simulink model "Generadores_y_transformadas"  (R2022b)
settings: Solver=ode4  StartTime=0.0  StopTime=0.1  FixedStep=1e-6  RelTol=1e-3
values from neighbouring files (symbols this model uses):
  f_AC = 60    [Generadores_y_tranformadas.m]
  Fase_A = 0    [Generadores_y_tranformadas.m]
  Fase_B = -120    [Generadores_y_tranformadas.m]
  Fase_C = 120    [Generadores_y_tranformadas.m]
  L_1 = 4.1e-3    (= 0.0041)    [Generadores_y_tranformadas.m]    (also in LQR_Sin_Integral.m; LQR_Con_Integral.m; Modal_Integral.m; Sistema_no_lineal_Modal.m)
  L_2 = 5.3e-3    (= 0.0053)    [Generadores_y_tranformadas.m]    (also in Sistema_no_lineal_Modal.m; Sistema_no_lineal_LQR.m; Sistema_control_no_lineal_LQR.m; Sistema_control_no_lineal_Modal.m)
  R_1 = 284e-3    (= 0.284)    [Generadores_y_tranformadas.m]    (also in LQR_Sin_Integral.m; LQR_Con_Integral.m; Modal_Integral.m; Sistema_no_lineal_Modal.m)
  R_2 = 330e-3    (= 0.33)    [Generadores_y_tranformadas.m]    (also in Sistema_no_lineal_Modal.m; Sistema_no_lineal_LQR.m; Sistema_control_no_lineal_LQR.m; Sistema_control_no_lineal_Modal.m)
  v_pico = v_RMS*sqrt(2)    [Generadores_y_tranformadas.m]
libraries: spsACVoltageSourceLib x6, spsGroundLib x6, spsCurrentMeasurementLib x6, spsVoltageMeasurementLib x6, spsSeriesRLCBranchLib x6, spsAlphaBetaZerotodq0Lib x4, spsabctoAlphaBetaZeroLib x4, spsAlphaBetaZerotoabcLib x1, spsdq0toAlphaBetaZeroLib x1, spspowerguiLib x1

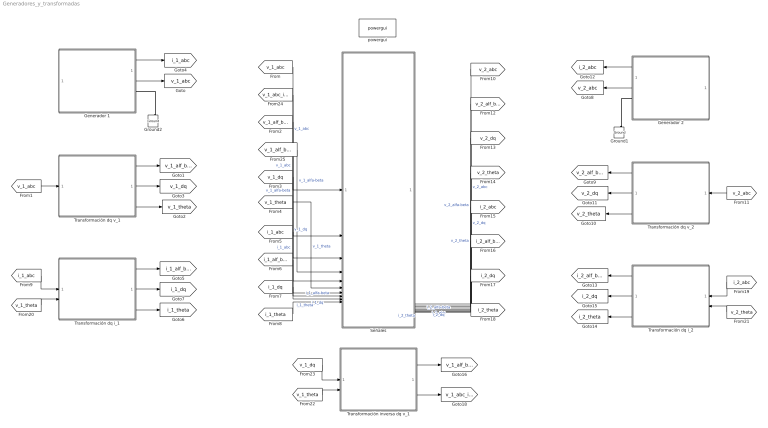
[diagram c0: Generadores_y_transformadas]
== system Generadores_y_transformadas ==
  Generador 1 : Subsystem
  Generador 2 : Subsystem
  Ground1 : spsGroundLib/Ground  LConnTagsString=a
  Ground2 : spsGroundLib/Ground  LConnTagsString=a
  Señales : Subsystem
  Transformación dq i_1 : Subsystem
  Transformación dq i_2 : Subsystem
  Transformación dq v_1 : Subsystem
  Transformación dq v_2 : Subsystem
  Transformación inversa dq v_1 : Subsystem
  powergui : spspowerguiLib/powergui  Priority=1  SimulationMode=Continuous  SampleTime=5e-6  frequency=Frecuencia_fuente  Iterations=50  frequencyindice=60  Pbase=100e6  ErrMax=1e-4  UnitsV=kV  UnitsW=MW  buscounter=0  FunctionMessages=off  echomessages=off  EnableUseOfTLC=off  CurrentSourceSwitches=off  DisableSnubberDevices=off  DisableRonSwitches=off  DisableVfSwitches=off  DisplayEquations=off  AutomaticDiscreteSolvers=off  SolverType=Tustin/Backward Euler (TBE)  Interpol=off  ExternalGateDelay=off  methode=off  Ts=100  x0status=blocks  SPID=on  SwTol=0  HookPort=off  NonlinearTolerance=1e-4  nMaxIteration=100  ContinueOnMaxIteration=off  RestoreLinks=warning  ResistiveCurrentMeasurement=off  Frange=[0:2:500]  Ylog=off  Xlog=on  ShowGrid=off  save=off  variable=ZData  structure=0  ZoomFFT=off  StartTime=0.0  cycles=1  DisplayStyle=1  fundamental=60  FreqAxis=off  MaxFrequency=1000  frequencyindicesteady=1  RmsSteady=1  display=off
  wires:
  Transformación dq i_1/1(i_1_alfa-beta) -> [i_1_alf_bet]
  Transformación dq i_1/3(Ángulo theta i_1) -> [i_1_theta]
  Transformación dq i_1/2(i_1_dq) -> [i_1_dq]
  Transformación dq v_1/1(v_1_alfa-beta) -> [v_1_alf_bet]
  [v_1_abc] -> Transformación dq v_1/1(v_1_abc)
  Transformación dq v_1/3(Ángulo theta v_1) -> [v_1_theta]
  Transformación dq v_1/2(v_1_dq) -> [v_1_dq]
  [i_1_abc] -> Transformación dq i_1/1(i_1_abc)
  Generador 1/1(i_1_abc) -> [i_1_abc]
  Generador 1/2(v_1_abc) -> [v_1_abc]
  [v_1_abc] -> Señales/1(v_1_abc)  "v_1_abc"
  [v_1_alf_bet] -> Señales/3(v_1_alfa-beta)  "v_1_alfa-beta"
  [v_1_dq] -> Señales/5(v_1_dq)  "v_1_dq"
  [v_1_theta] -> Señales/6(v_1_theta)  "v_1_theta"
  [i_1_abc] -> Señales/7(i_1_abc)  "i_1_abc"
  [i_1_alf_bet] -> Señales/8(i_1_alfa-beta)  "i_1_alfa-beta"
  [i_1_dq] -> Señales/9(i_1_dq)  "i_1_dq"
  [i_1_theta] -> Señales/10(i_1_theta)  "i_1_theta"
  Generador 2/2(v_2_abc) -> [v_2_abc]
  Generador 2/1(i_2_abc) -> [i_2_abc]
  [i_2_abc] -> Transformación dq i_2/1(i_2_abc)
  Transformación dq v_2/2(v_2_dq) -> [v_2_dq]
  Transformación dq v_2/3(Ángulo theta v_2) -> [v_2_theta]
  [v_2_abc] -> Transformación dq v_2/1(v_2_abc)
  Transformación dq v_2/1(v_2_alfa-beta) -> [v_2_alf_bet]
  Transformación dq i_2/2(i_2_dq) -> [i_2_dq]
  Transformación dq i_2/3(Ángulo theta i_2) -> [i_2_theta]
  Transformación dq i_2/1(i_2_alfa-beta) -> [i_2_alf_bet]
  [v_2_abc] -> Señales/11(v_2_abc)  "v_2_abc"
  [v_2_alf_bet] -> Señales/12(v_2_alfa-beta)  "v_2_alfa-beta"
  [v_2_dq] -> Señales/13(v_2_dq)  "v_2_dq"
  [v_2_theta] -> Señales/14(v_2_theta)  "v_2_theta"
  [i_2_abc] -> Señales/15(i_2_abc)  "i_2_abc"
  [i_2_alf_bet] -> Señales/16(i_2_alfa-beta)  "i_2_alfa-beta"
  [i_2_dq] -> Señales/17(i_2_dq)  "i_2_dq"
  [i_2_theta] -> Señales/18(i_2_theta)  "i_2_theta"
  [v_1_theta] -> Transformación dq i_1/2(Ángulo theta v_1)
  [v_2_theta] -> Transformación dq i_2/2(Ángulo theta v_2)
  [v_1_dq] -> Transformación inversa dq v_1/1(v_1_dq)
  Transformación inversa dq v_1/2(v_1_abc) -> [v_1_abc_inv]
  [v_1_theta] -> Transformación inversa dq v_1/2(Ángulo theta v_1)
  Transformación inversa dq v_1/1(v_1_alfa-beta) -> [v_1_alf_bet_inv]
  [v_1_abc_inv] -> Señales/2(v_1_abc_inv)  "v_1_abc"
  [v_1_alf_bet_inv] -> Señales/4(v_1_alfa-beta_inv)  "v_1_alfa-beta"
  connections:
  Ground2/LConn1 -- Generador 1/RConn1
  Ground1/LConn1 -- Generador 2/RConn1

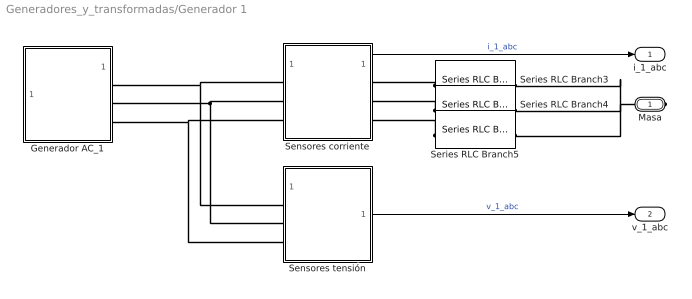
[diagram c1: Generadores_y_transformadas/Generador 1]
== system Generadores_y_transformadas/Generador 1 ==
  Generador AC_1 : Subsystem
  Sensores corriente : Subsystem
  Sensores tensión : Subsystem
  Series RLC Branch3 : spsSeriesRLCBranchLib/Series RLC Branch  LConnTagsString=__new0  RConnTagsString=__new0  BranchType=RL  Resistance=R_1  Inductance=L_1  SetiL0=off  InitialCurrent=0  Capacitance=1e-6  Setx0=off  InitialVoltage=0  Measurements=None
  Series RLC Branch4 : spsSeriesRLCBranchLib/Series RLC Branch  LConnTagsString=__new0  RConnTagsString=__new0  BranchType=RL  Resistance=R_1  Inductance=L_1  SetiL0=off  InitialCurrent=0  Capacitance=1e-6  Setx0=off  InitialVoltage=0  Measurements=None
  Series RLC Branch5 : spsSeriesRLCBranchLib/Series RLC Branch  LConnTagsString=__new0  RConnTagsString=__new0  BranchType=RL  Resistance=R_1  Inductance=L_1  SetiL0=off  InitialCurrent=0  Capacitance=1e-6  Setx0=off  InitialVoltage=0  Measurements=None
  Masa : PMIOPort  Side=Right
  i_1_abc : Outport
  v_1_abc : Outport  Port=2
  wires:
  Sensores tensión/1(v_1_abc) -> v_1_abc/1  "v_1_abc"
  Sensores corriente/1(i_1_abc) -> i_1_abc/1  "i_1_abc"
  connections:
  Masa/RConn1 -- Series RLC Branch5/RConn1 -- Series RLC Branch4/RConn1 -- Series RLC Branch3/RConn1
  Sensores tensión/LConn2 -- Generador AC_1/RConn2 -- Sensores corriente/LConn2
  Generador AC_1/RConn1 -- Sensores corriente/LConn1 -- Sensores tensión/LConn1
  Sensores tensión/LConn3 -- Generador AC_1/RConn3 -- Sensores corriente/LConn3
  Series RLC Branch4/LConn1 -- Sensores corriente/RConn2
  Series RLC Branch3/LConn1 -- Sensores corriente/RConn1
  Series RLC Branch5/LConn1 -- Sensores corriente/RConn3

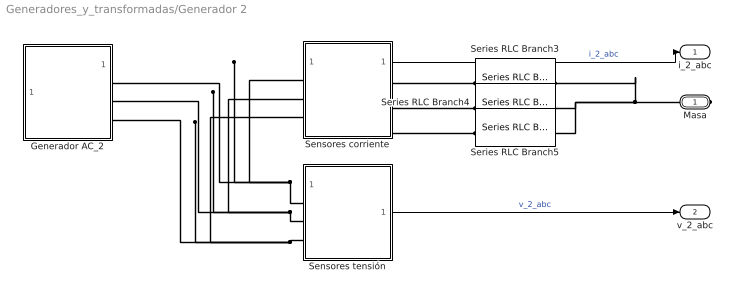
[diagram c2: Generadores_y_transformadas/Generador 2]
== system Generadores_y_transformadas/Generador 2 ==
  Generador AC_2 : Subsystem
  Sensores corriente : Subsystem
  Sensores tensión : Subsystem
  Series RLC Branch3 : spsSeriesRLCBranchLib/Series RLC Branch  LConnTagsString=__new0  RConnTagsString=__new0  BranchType=RL  Resistance=R_2  Inductance=L_2  SetiL0=off  InitialCurrent=0  Capacitance=1e-6  Setx0=off  InitialVoltage=0  Measurements=None
  Series RLC Branch4 : spsSeriesRLCBranchLib/Series RLC Branch  LConnTagsString=__new0  RConnTagsString=__new0  BranchType=RL  Resistance=R_2  Inductance=L_2  SetiL0=off  InitialCurrent=0  Capacitance=1e-6  Setx0=off  InitialVoltage=0  Measurements=None
  Series RLC Branch5 : spsSeriesRLCBranchLib/Series RLC Branch  LConnTagsString=__new0  RConnTagsString=__new0  BranchType=RL  Resistance=R_2  Inductance=L_2  SetiL0=off  InitialCurrent=0  Capacitance=1e-6  Setx0=off  InitialVoltage=0  Measurements=None
  Masa : PMIOPort  Side=Right
  i_2_abc : Outport
  v_2_abc : Outport  Port=2
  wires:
  Sensores corriente/1(i_2_abc) -> i_2_abc/1  "i_2_abc"
  Sensores tensión/1(v_2_abc) -> v_2_abc/1  "v_2_abc"
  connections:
  Sensores tensión/LConn1 -- Generador AC_2/RConn1 -- Sensores corriente/LConn1
  Sensores tensión/LConn3 -- Generador AC_2/RConn3 -- Sensores corriente/LConn3
  Sensores corriente/RConn3 -- Series RLC Branch5/LConn1
  Sensores corriente/RConn2 -- Series RLC Branch4/LConn1
  Sensores corriente/RConn1 -- Series RLC Branch3/LConn1
  Masa/RConn1 -- Series RLC Branch5/RConn1 -- Series RLC Branch3/RConn1 -- Series RLC Branch4/RConn1
  Sensores tensión/LConn2 -- Generador AC_2/RConn2 -- Sensores corriente/LConn2

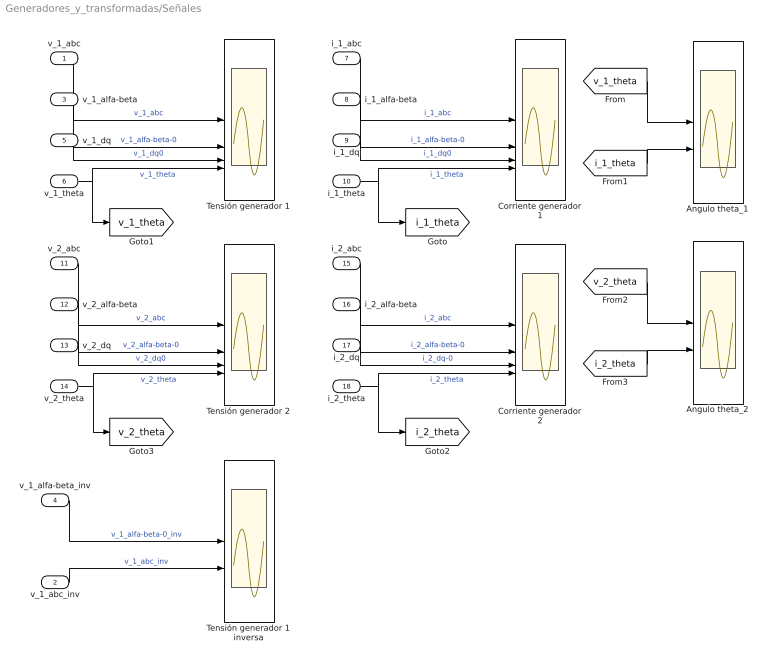
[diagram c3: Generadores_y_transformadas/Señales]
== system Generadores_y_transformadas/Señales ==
  v_1_abc : Inport
  v_1_abc_inv : Inport  Port=2
  v_1_alfa-beta : Inport  Port=3
  v_1_alfa-beta_inv : Inport  Port=4
  v_1_dq : Inport  Port=5
  v_1_theta : Inport  Port=6
  i_1_abc : Inport  Port=7
  i_1_alfa-beta : Inport  Port=8
  i_1_dq : Inport  Port=9
  i_1_theta : Inport  Port=10
  v_2_abc : Inport  Port=11
  v_2_alfa-beta : Inport  Port=12
  v_2_dq : Inport  Port=13
  v_2_theta : Inport  Port=14
  i_2_abc : Inport  Port=15
  i_2_alfa-beta : Inport  Port=16
  i_2_dq : Inport  Port=17
  i_2_theta : Inport  Port=18
  Angulo theta_1 : Scope  NumInputPorts=2
  Angulo theta_2 : Scope  NumInputPorts=2
  Corriente generador 1 : Scope  NumInputPorts=4
  Corriente generador 2 : Scope  NumInputPorts=4
  Tensión generador 1 : Scope  NumInputPorts=4
  Tensión generador 1 inversa : Scope  NumInputPorts=2
  Tensión generador 2 : Scope  NumInputPorts=4
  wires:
  v_1_alfa-beta/1 -> Tensión generador 1/2  "v_1_alfa-beta-0"
  v_1_theta/1 -> Tensión generador 1/4, [v_1_theta]  "v_1_theta"
  v_1_dq/1 -> Tensión generador 1/3  "v_1_dq0"
  v_1_abc/1 -> Tensión generador 1/1  "v_1_abc"
  i_1_abc/1 -> Corriente generador 1/1  "i_1_abc"
  i_1_dq/1 -> Corriente generador 1/3  "i_1_dq0"
  i_1_theta/1 -> Corriente generador 1/4, [i_1_theta]  "i_1_theta"
  i_1_alfa-beta/1 -> Corriente generador 1/2  "i_1_alfa-beta-0"
  v_2_abc/1 -> Tensión generador 2/1  "v_2_abc"
  v_2_alfa-beta/1 -> Tensión generador 2/2  "v_2_alfa-beta-0"
  v_2_dq/1 -> Tensión generador 2/3  "v_2_dq0"
  v_2_theta/1 -> Tensión generador 2/4, [v_2_theta]  "v_2_theta"
  i_2_theta/1 -> Corriente generador 2/4, [i_2_theta]  "i_2_theta"
  i_2_dq/1 -> Corriente generador 2/3  "i_2_dq-0"
  i_2_alfa-beta/1 -> Corriente generador 2/2  "i_2_alfa-beta-0"
  i_2_abc/1 -> Corriente generador 2/1  "i_2_abc"
  [v_1_theta] -> Angulo theta_1/1
  [i_1_theta] -> Angulo theta_1/2
  [i_2_theta] -> Angulo theta_2/2
  [v_2_theta] -> Angulo theta_2/1
  v_1_alfa-beta_inv/1 -> Tensión generador 1 inversa/1  "v_1_alfa-beta-0_inv"
  v_1_abc_inv/1 -> Tensión generador 1 inversa/2  "v_1_abc_inv"

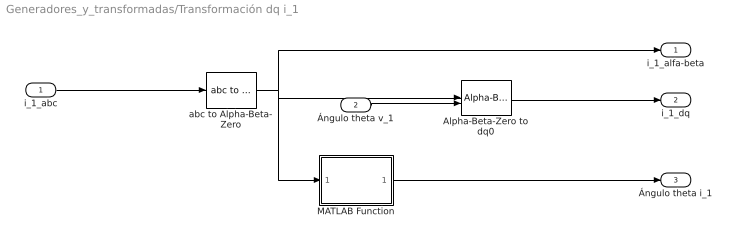
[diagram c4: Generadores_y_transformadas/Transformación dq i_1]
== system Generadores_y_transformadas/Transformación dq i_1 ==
  i_1_abc : Inport
  Ángulo theta v_1 : Inport  Port=2
  Alpha-Beta-Zero to dq0 : spsAlphaBetaZerotodq0Lib/Alpha-Beta-Zero to dq0  Alignment=Aligned with phase A axis
  MATLAB Function : MATLAB Function  TreatAsAtomicUnit=on
  abc to Alpha-Beta-Zero : spsabctoAlphaBetaZeroLib/abc to Alpha-Beta-Zero
  i_1_alfa-beta : Outport
  i_1_dq : Outport  Port=2
  Ángulo theta i_1 : Outport  Port=3
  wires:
  i_1_abc/1 -> abc to Alpha-Beta-Zero/1
  MATLAB Function/1(angulo) -> Ángulo theta i_1/1
  Alpha-Beta-Zero to dq0/1 -> i_1_dq/1
  abc to Alpha-Beta-Zero/1 -> i_1_alfa-beta/1, Alpha-Beta-Zero to dq0/1, MATLAB Function/1(u)
  Ángulo theta v_1/1 -> Alpha-Beta-Zero to dq0/2

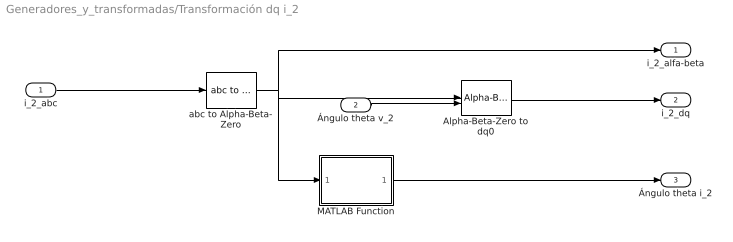
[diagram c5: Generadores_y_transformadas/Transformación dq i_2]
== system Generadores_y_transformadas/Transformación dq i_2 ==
  i_2_abc : Inport
  Ángulo theta v_2 : Inport  Port=2
  Alpha-Beta-Zero to dq0 : spsAlphaBetaZerotodq0Lib/Alpha-Beta-Zero to dq0  Alignment=Aligned with phase A axis
  MATLAB Function : MATLAB Function  TreatAsAtomicUnit=on
  abc to Alpha-Beta-Zero : spsabctoAlphaBetaZeroLib/abc to Alpha-Beta-Zero
  i_2_alfa-beta : Outport
  i_2_dq : Outport  Port=2
  Ángulo theta i_2 : Outport  Port=3
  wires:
  abc to Alpha-Beta-Zero/1 -> MATLAB Function/1(u), Alpha-Beta-Zero to dq0/1, i_2_alfa-beta/1
  Alpha-Beta-Zero to dq0/1 -> i_2_dq/1
  MATLAB Function/1(angulo) -> Ángulo theta i_2/1
  i_2_abc/1 -> abc to Alpha-Beta-Zero/1
  Ángulo theta v_2/1 -> Alpha-Beta-Zero to dq0/2

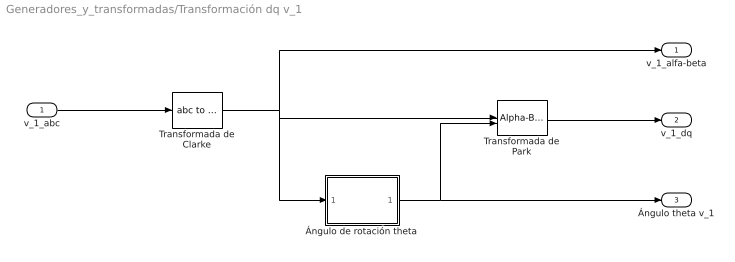
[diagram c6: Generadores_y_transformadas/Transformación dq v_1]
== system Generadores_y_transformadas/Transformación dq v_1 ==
  v_1_abc : Inport
  Transformada de Clarke : spsabctoAlphaBetaZeroLib/abc to Alpha-Beta-Zero
  Transformada de Park : spsAlphaBetaZerotodq0Lib/Alpha-Beta-Zero to dq0  Alignment=Aligned with phase A axis
  Ángulo de rotación theta : MATLAB Function  TreatAsAtomicUnit=on
  v_1_alfa-beta : Outport
  v_1_dq : Outport  Port=2
  Ángulo theta v_1 : Outport  Port=3
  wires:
  v_1_abc/1 -> Transformada de Clarke/1
  Ángulo de rotación theta/1(angulo) -> Ángulo theta v_1/1, Transformada de Park/2
  Transformada de Park/1 -> v_1_dq/1
  Transformada de Clarke/1 -> v_1_alfa-beta/1, Transformada de Park/1, Ángulo de rotación theta/1(u)

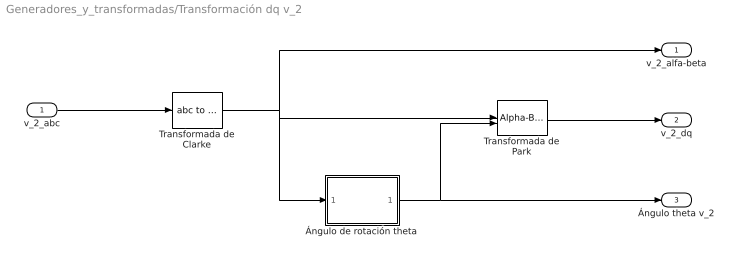
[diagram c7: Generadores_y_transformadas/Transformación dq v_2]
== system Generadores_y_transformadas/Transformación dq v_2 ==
  v_2_abc : Inport
  Transformada de Clarke : spsabctoAlphaBetaZeroLib/abc to Alpha-Beta-Zero
  Transformada de Park : spsAlphaBetaZerotodq0Lib/Alpha-Beta-Zero to dq0  Alignment=Aligned with phase A axis
  Ángulo de rotación theta : MATLAB Function  TreatAsAtomicUnit=on
  v_2_alfa-beta : Outport
  v_2_dq : Outport  Port=2
  Ángulo theta v_2 : Outport  Port=3
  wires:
  Transformada de Clarke/1 -> Ángulo de rotación theta/1(u), Transformada de Park/1, v_2_alfa-beta/1
  Transformada de Park/1 -> v_2_dq/1
  Ángulo de rotación theta/1(angulo) -> Transformada de Park/2, Ángulo theta v_2/1
  v_2_abc/1 -> Transformada de Clarke/1

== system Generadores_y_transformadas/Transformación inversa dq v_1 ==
  v_1_dq : Inport
  Ángulo theta v_1 : Inport  Port=2
  Alpha-Beta-Zero to abc : spsAlphaBetaZerotoabcLib/Alpha-Beta-Zero to abc
  dq0 to Alpha-Beta-Zero : spsdq0toAlphaBetaZeroLib/dq0 to Alpha-Beta-Zero  Alignment=90 degrees behind phase A axis
  v_1_alfa-beta : Outport
  v_1_abc : Outport  Port=2
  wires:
  v_1_dq/1 -> dq0 to Alpha-Beta-Zero/1
  Alpha-Beta-Zero to abc/1 -> v_1_abc/1
  dq0 to Alpha-Beta-Zero/1 -> v_1_alfa-beta/1, Alpha-Beta-Zero to abc/1
  Ángulo theta v_1/1 -> dq0 to Alpha-Beta-Zero/2

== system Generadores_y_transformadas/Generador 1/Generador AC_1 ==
  Generador fase A : spsACVoltageSourceLib/AC Voltage Source  Amplitude=v_pico  Phase=Fase_A  Frequency=f_AC  SampleTime=0  Measurements=Voltage  BusType=swing  Pref=10e3  Qref=0  Qmin=-inf  Qmax=+inf
  Generador fase B : spsACVoltageSourceLib/AC Voltage Source  Amplitude=v_pico  Phase=Fase_B  Frequency=f_AC  SampleTime=0  Measurements=Voltage  BusType=swing  Pref=10e3  Qref=0  Qmin=-inf  Qmax=+inf
  Generador fase C : spsACVoltageSourceLib/AC Voltage Source  Amplitude=v_pico  Phase=Fase_C  Frequency=f_AC  SampleTime=0  Measurements=Voltage  BusType=swing  Pref=10e3  Qref=0  Qmin=-inf  Qmax=+inf
  Ground3 : spsGroundLib/Ground  LConnTagsString=a
  Fase A : PMIOPort  Side=Right
  Fase B : PMIOPort  Port=2  Side=Right
  Fase C : PMIOPort  Port=3  Side=Right
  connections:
  Generador fase C/RConn1 -- Fase C/RConn1
  Generador fase B/RConn1 -- Fase B/RConn1
  Generador fase A/RConn1 -- Fase A/RConn1
  Generador fase B/LConn1 -- Generador fase C/LConn1 -- Ground3/LConn1 -- Generador fase A/LConn1

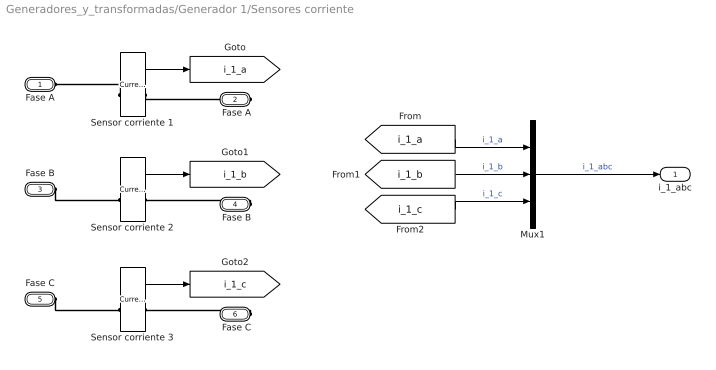
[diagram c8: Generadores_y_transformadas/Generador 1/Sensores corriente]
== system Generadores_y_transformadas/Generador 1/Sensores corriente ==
  Mux1 : Mux  Inputs=3
  Sensor corriente 1 : spsCurrentMeasurementLib/Current Measurement  PhasorSimulation=off  OutputType=Complex  PSBequivalent=0
  Sensor corriente 2 : spsCurrentMeasurementLib/Current Measurement  PhasorSimulation=off  OutputType=Complex  PSBequivalent=0
  Sensor corriente 3 : spsCurrentMeasurementLib/Current Measurement  PhasorSimulation=off  OutputType=Complex  PSBequivalent=0
  Fase A : PMIOPort  Side=Left
  " Fase A" : PMIOPort  Port=2  Side=Right
  Fase B : PMIOPort  Port=3  Side=Left
  " Fase B" : PMIOPort  Port=4  Side=Right
  Fase C : PMIOPort  Port=5  Side=Left
  " Fase C" : PMIOPort  Port=6  Side=Right
  i_1_abc : Outport
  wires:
  Mux1/1 -> i_1_abc/1  "i_1_abc"
  Sensor corriente 1/1 -> [i_1_a]
  [i_1_a] -> Mux1/1  "i_1_a"
  Sensor corriente 2/1 -> [i_1_b]
  [i_1_b] -> Mux1/2  "i_1_b"
  Sensor corriente 3/1 -> [i_1_c]
  [i_1_c] -> Mux1/3  "i_1_c"
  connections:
  Fase C/RConn1 -- Sensor corriente 3/LConn1
  " Fase B"/RConn1 -- Sensor corriente 2/RConn1
  Fase B/RConn1 -- Sensor corriente 2/LConn1
  Sensor corriente 1/LConn1 -- Fase A/RConn1
  " Fase C"/RConn1 -- Sensor corriente 3/RConn1
  Sensor corriente 1/RConn1 -- " Fase A"/RConn1

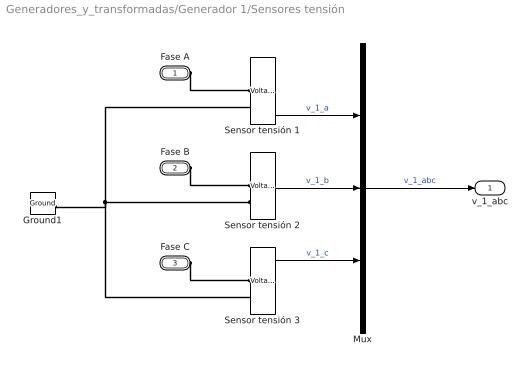
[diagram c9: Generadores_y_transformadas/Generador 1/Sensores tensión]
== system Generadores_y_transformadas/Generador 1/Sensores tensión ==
  Ground1 : spsGroundLib/Ground  LConnTagsString=a
  Mux : Mux  Inputs=3
  Sensor tensión 1 : spsVoltageMeasurementLib/Voltage Measurement  PhasorSimulation=off  OutputType=Complex  PSBequivalent=0
  Sensor tensión 2 : spsVoltageMeasurementLib/Voltage Measurement  PhasorSimulation=off  OutputType=Complex  PSBequivalent=0
  Sensor tensión 3 : spsVoltageMeasurementLib/Voltage Measurement  PhasorSimulation=off  OutputType=Complex  PSBequivalent=0
  Fase A : PMIOPort  Side=Left
  Fase B : PMIOPort  Port=2  Side=Left
  Fase C : PMIOPort  Port=3  Side=Left
  v_1_abc : Outport
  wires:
  Mux/1 -> v_1_abc/1  "v_1_abc"
  Sensor tensión 2/1 -> Mux/2  "v_1_b"
  Sensor tensión 3/1 -> Mux/3  "v_1_c"
  Sensor tensión 1/1 -> Mux/1  "v_1_a"
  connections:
  Fase B/RConn1 -- Sensor tensión 2/LConn1
  Fase C/RConn1 -- Sensor tensión 3/LConn1
  Fase A/RConn1 -- Sensor tensión 1/LConn1
  Sensor tensión 2/LConn2 -- Sensor tensión 1/LConn2 -- Ground1/LConn1 -- Sensor tensión 3/LConn2

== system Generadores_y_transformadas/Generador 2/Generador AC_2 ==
  Generador fase A : spsACVoltageSourceLib/AC Voltage Source  Amplitude=v_pico  Phase=Fase_A  Frequency=f_AC  SampleTime=0  Measurements=Voltage  BusType=swing  Pref=10e3  Qref=0  Qmin=-inf  Qmax=+inf
  Generador fase B : spsACVoltageSourceLib/AC Voltage Source  Amplitude=v_pico  Phase=Fase_B  Frequency=f_AC  SampleTime=0  Measurements=Voltage  BusType=swing  Pref=10e3  Qref=0  Qmin=-inf  Qmax=+inf
  Generador fase C : spsACVoltageSourceLib/AC Voltage Source  Amplitude=v_pico  Phase=Fase_C  Frequency=f_AC  SampleTime=0  Measurements=Voltage  BusType=swing  Pref=10e3  Qref=0  Qmin=-inf  Qmax=+inf
  Ground3 : spsGroundLib/Ground  LConnTagsString=a
  Fase A : PMIOPort  Side=Right
  Fase B : PMIOPort  Port=2  Side=Right
  Fase C : PMIOPort  Port=3  Side=Right
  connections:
  Ground3/LConn1 -- Generador fase A/LConn1 -- Generador fase B/LConn1 -- Generador fase C/LConn1
  Generador fase A/RConn1 -- Fase A/RConn1
  Generador fase B/RConn1 -- Fase B/RConn1
  Generador fase C/RConn1 -- Fase C/RConn1

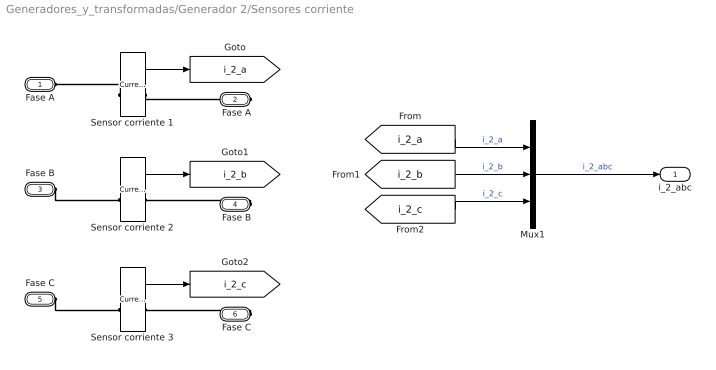
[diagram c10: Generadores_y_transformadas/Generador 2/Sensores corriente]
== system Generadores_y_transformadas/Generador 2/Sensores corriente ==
  Mux1 : Mux  Inputs=3
  Sensor corriente 1 : spsCurrentMeasurementLib/Current Measurement  PhasorSimulation=off  OutputType=Complex  PSBequivalent=0
  Sensor corriente 2 : spsCurrentMeasurementLib/Current Measurement  PhasorSimulation=off  OutputType=Complex  PSBequivalent=0
  Sensor corriente 3 : spsCurrentMeasurementLib/Current Measurement  PhasorSimulation=off  OutputType=Complex  PSBequivalent=0
  Fase A : PMIOPort  Side=Left
  " Fase A" : PMIOPort  Port=2  Side=Right
  Fase B : PMIOPort  Port=3  Side=Left
  " Fase B" : PMIOPort  Port=4  Side=Right
  Fase C : PMIOPort  Port=5  Side=Left
  " Fase C" : PMIOPort  Port=6  Side=Right
  i_2_abc : Outport
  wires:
  [i_2_c] -> Mux1/3  "i_2_c"
  Sensor corriente 3/1 -> [i_2_c]
  [i_2_b] -> Mux1/2  "i_2_b"
  Sensor corriente 2/1 -> [i_2_b]
  [i_2_a] -> Mux1/1  "i_2_a"
  Sensor corriente 1/1 -> [i_2_a]
  Mux1/1 -> i_2_abc/1  "i_2_abc"
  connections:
  Sensor corriente 1/RConn1 -- " Fase A"/RConn1
  " Fase C"/RConn1 -- Sensor corriente 3/RConn1
  Sensor corriente 1/LConn1 -- Fase A/RConn1
  Fase B/RConn1 -- Sensor corriente 2/LConn1
  " Fase B"/RConn1 -- Sensor corriente 2/RConn1
  Fase C/RConn1 -- Sensor corriente 3/LConn1

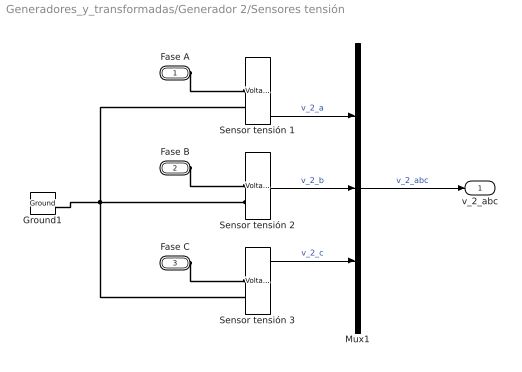
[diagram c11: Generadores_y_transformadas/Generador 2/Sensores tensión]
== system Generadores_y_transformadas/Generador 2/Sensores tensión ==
  Ground1 : spsGroundLib/Ground  LConnTagsString=a
  Mux1 : Mux  Inputs=3
  Sensor tensión 1 : spsVoltageMeasurementLib/Voltage Measurement  PhasorSimulation=off  OutputType=Complex  PSBequivalent=0
  Sensor tensión 2 : spsVoltageMeasurementLib/Voltage Measurement  PhasorSimulation=off  OutputType=Complex  PSBequivalent=0
  Sensor tensión 3 : spsVoltageMeasurementLib/Voltage Measurement  PhasorSimulation=off  OutputType=Complex  PSBequivalent=0
  Fase A : PMIOPort  Side=Left
  Fase B : PMIOPort  Port=2  Side=Left
  Fase C : PMIOPort  Port=3  Side=Left
  v_2_abc : Outport
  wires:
  Sensor tensión 3/1 -> Mux1/3  "v_2_c"
  Sensor tensión 2/1 -> Mux1/2  "v_2_b"
  Sensor tensión 1/1 -> Mux1/1  "v_2_a"
  Mux1/1 -> v_2_abc/1  "v_2_abc"
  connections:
  Sensor tensión 2/LConn2 -- Ground1/LConn1 -- Sensor tensión 1/LConn2 -- Sensor tensión 3/LConn2
  Fase A/RConn1 -- Sensor tensión 1/LConn1
  Fase B/RConn1 -- Sensor tensión 2/LConn1
  Fase C/RConn1 -- Sensor tensión 3/LConn1

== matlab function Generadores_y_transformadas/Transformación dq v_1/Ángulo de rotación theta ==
function angulo = fcn(u)

angulo = atan2(u(2),u(1));

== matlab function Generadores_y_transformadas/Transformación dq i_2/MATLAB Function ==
function angulo = fcn(u)

angulo = atan2(u(2),u(1));

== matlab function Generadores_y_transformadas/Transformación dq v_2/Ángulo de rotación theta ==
function angulo = fcn(u)

angulo = atan2(u(2),u(1));

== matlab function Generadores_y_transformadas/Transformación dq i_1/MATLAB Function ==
function angulo = fcn(u)

angulo = atan2(u(2),u(1));
